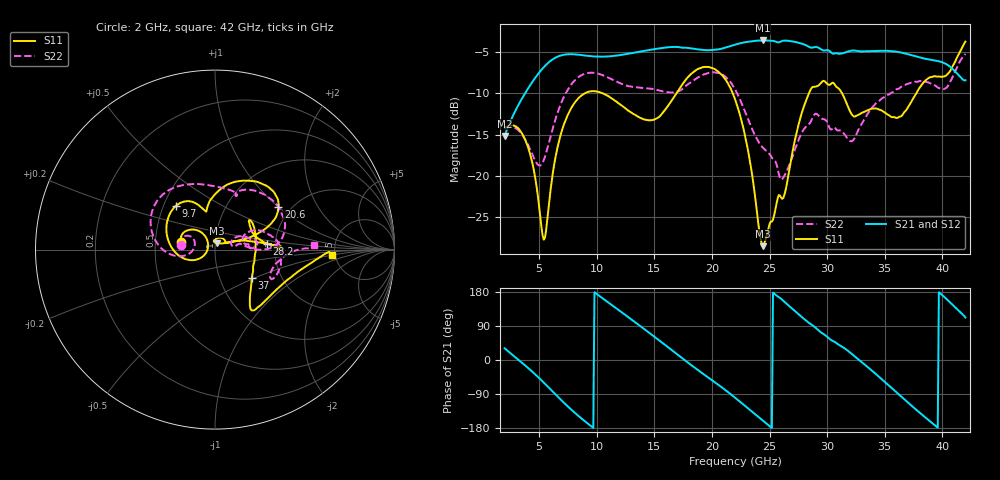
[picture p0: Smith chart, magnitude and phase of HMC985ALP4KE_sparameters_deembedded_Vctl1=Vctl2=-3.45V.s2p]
!s2p File: Measurements: S11, S21, S12, S22
# GHz S dB R 50.0
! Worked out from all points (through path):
!   401 points, 2 GHz to 42 GHz, reference 50 ohm
!   highest |S21| = -3.55 dB at 24.4 GHz (marker M1); lowest = -15.2 dB at 2 GHz (marker M2)
!   lowest |S11| = -28.6 dB at 24.4 GHz (marker M3), VSWR 1.08, Z = 50.9 + j3.66 ohm
!   |S11| at or under -10 dB: start of sweep to 8.938 GHz; 21.81 GHz to 28.41 GHz (6.603 GHz wide, 26.3 % of centre); 31.3 GHz to 37.73 GHz (6.428 GHz wide, 18.6 % of centre)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
!   |S22| runs from -20.5 to -5.2 dB; largest |S21 - S12| = 0.00075
!   S11 on the Smith chart (normalised r, x): 2 GHz: 0.68, +0.06; 9.7 GHz: 0.58, +0.31; 20.6 GHz: 1.73, +1.00; 28.2 GHz: 1.80, +0.13; 37 GHz: 1.42, -0.48; 42 GHz: 4.71, -0.53
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2  -14.15 167.7  -15.18 30.9  -15.17 30.8  -14.31 172.3
3.9  -16.02 135.5  -9.70 -17.4  -9.70 -17.4  -15.86 152.1
5.4  -27.77 166.4  -6.80 -59.5  -6.80 -59.5  -18.10 -178.1
6.8  -15.36 -161.7  -5.42 -102.3  -5.42 -102.3  -11.56 -175.9
8.7  -10.21 149.9  -5.34 -155.0  -5.34 -155.0  -7.76 149.1
9.7  -9.71 132.3  -5.49 -179.0  -5.49 -179.0  -7.48 132.7
12.9  -12.23 107.5  -5.13 109.4  -5.13 109.4  -9.14 86.6
15.4  -12.86 101.6  -4.53 52.2  -4.53 52.2  -9.62 68.1
17.8  -8.20 74.6  -4.45 -4.2  -4.45 -4.2  -9.01 67.5
20.6  -7.41 33.9  -4.63 -66.5  -4.63 -66.5  -7.52 24.2
22  -10.67 22.0  -4.07 -99.4  -4.07 -99.4  -9.49 3.8
24.4  -28.56 74.1  -3.56 -159.2  -3.56 -159.3  -16.56 11.9
26.1  -22.81 33.3  -3.61 158.9  -3.62 158.9  -20.40 21.4
28.2  -10.75 6.7  -4.16 103.2  -4.16 103.1  -13.99 18.0
28.7  -9.25 0.7  -4.43 92.3  -4.44 92.3  -13.03 15.0
30.6  -8.79 1.8  -5.16 48.8  -5.16 48.8  -14.09 7.9
32.4  -12.80 27.1  -4.79 9.2  -4.79 9.2  -15.37 24.1
33.9  -11.84 39.3  -4.86 -28.5  -4.86 -28.5  -11.71 24.8
35.4  -12.67 12.1  -4.83 -68.6  -4.83 -68.6  -10.09 15.2
37  -11.72 -37.6  -5.22 -111.9  -5.22 -111.9  -8.83 2.7
39.6  -7.95 -52.9  -6.05 -178.6  -6.05 -178.6  -9.28 -26.9
42  -3.70 -2.8  -8.39 111.9  -8.39 111.9  -5.19 2.8
